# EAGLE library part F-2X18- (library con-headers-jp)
FEMALE HEADER
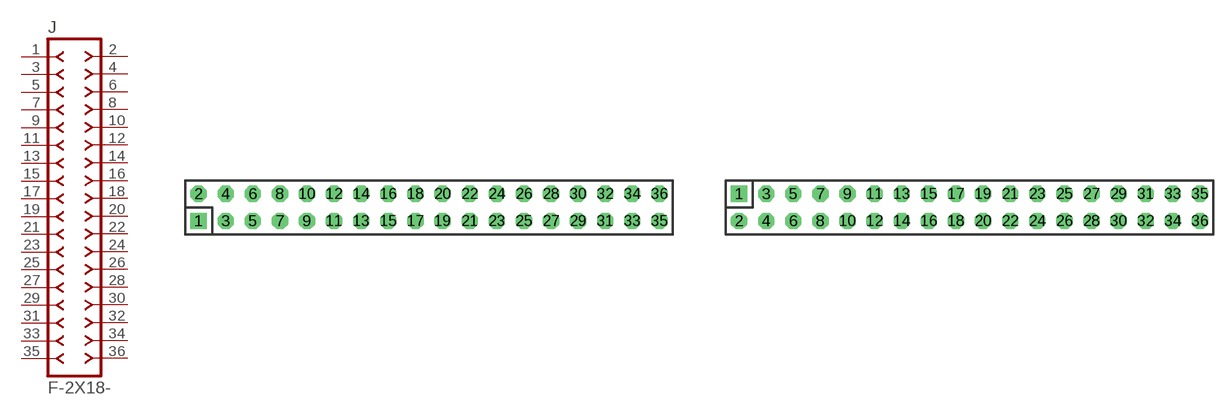
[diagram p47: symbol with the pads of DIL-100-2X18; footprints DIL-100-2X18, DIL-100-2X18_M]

Designator prefix J

## F-2X18-DIL-100  [DIL-100-2X18]
1  1  pas
2  2  pas
3  3  pas
4  4  pas
5  5  pas
6  6  pas
7  7  pas
8  8  pas
9  9  pas
10  10  pas
11  11  pas
12  12  pas
13  13  pas
14  14  pas
15  15  pas
16  16  pas
17  17  pas
18  18  pas
19  19  pas
20  20  pas
21  21  pas
22  22  pas
23  23  pas
24  24  pas
25  25  pas
26  26  pas
27  27  pas
28  28  pas
29  29  pas
30  30  pas
31  31  pas
32  32  pas
33  33  pas
34  34  pas
35  35  pas
36  36  pas

## F-2X18-DIL-100_M  [DIL-100-2X18_M]
Pads as for DIL-100-2X18

## F-2X18-DIL-2MM  [DIL-2MM-2X18]
Pads as for DIL-100-2X18

## F-2X18-DIL-2MM_M  [DIL-2MM-2X18_M]
Pads as for DIL-100-2X18

## F-2X18-71991  [71991-36]
Pads as for DIL-100-2X18

## Footprint DIL-100-2X18 (pad centres in mm)
PIN HEADER - 0.1"
drill 1.016 square: 1 -21.59,-1.27
drill 1.016 octagon: 2 -21.59,1.27; 3 -19.05,-1.27; 4 -19.05,1.27; 5 -16.51,-1.27; 6 -16.51,1.27; 7 -13.97,-1.27; 8 -13.97,1.27; 9 -11.43,-1.27; 10 -11.43,1.27; 11 -8.89,-1.27; 12 -8.89,1.27; 13 -6.35,-1.27; 14 -6.35,1.27; 15 -3.81,-1.27; 16 -3.81,1.27; 17 -1.27,-1.27; 18 -1.27,1.27; 19 1.27,-1.27; 20 1.27,1.27; 21 3.81,-1.27; 22 3.81,1.27; 23 6.35,-1.27; 24 6.35,1.27; 25 8.89,-1.27; 26 8.89,1.27; 27 11.43,-1.27; 28 11.43,1.27; 29 13.97,-1.27; 30 13.97,1.27; 31 16.51,-1.27; 32 16.51,1.27; 33 19.05,-1.27; 34 19.05,1.27; 35 21.59,-1.27; 36 21.59,1.27

## Footprint DIL-100-2X18_M (pad centres in mm)
PIN HEADER - MIRRORED 0.1"
drill 1.016 square: 1 -21.59,1.27
drill 1.016 octagon: 2 -21.59,-1.27; 3 -19.05,1.27; 4 -19.05,-1.27; 5 -16.51,1.27; 6 -16.51,-1.27; 7 -13.97,1.27; 8 -13.97,-1.27; 9 -11.43,1.27; 10 -11.43,-1.27; 11 -8.89,1.27; 12 -8.89,-1.27; 13 -6.35,1.27; 14 -6.35,-1.27; 15 -3.81,1.27; 16 -3.81,-1.27; 17 -1.27,1.27; 18 -1.27,-1.27; 19 1.27,1.27; 20 1.27,-1.27; 21 3.81,1.27; 22 3.81,-1.27; 23 6.35,1.27; 24 6.35,-1.27; 25 8.89,1.27; 26 8.89,-1.27; 27 11.43,1.27; 28 11.43,-1.27; 29 13.97,1.27; 30 13.97,-1.27; 31 16.51,1.27; 32 16.51,-1.27; 33 19.05,1.27; 34 19.05,-1.27; 35 21.59,1.27; 36 21.59,-1.27

## Footprint DIL-2MM-2X18 (pad centres in mm)
PIN HEADER - 2MM
drill 0.711 square: 1 -17,-1
drill 0.711: 2 -17,1; 3 -15,-1; 4 -15,1; 5 -13,-1; 6 -13,1; 7 -11,-1; 8 -11,1; 9 -9,-1; 10 -9,1; 11 -7,-1; 12 -7,1; 13 -5,-1; 14 -5,1; 15 -3,-1; 16 -3,1; 17 -1,-1; 18 -1,1; 19 1,-1; 20 1,1; 21 3,-1; 22 3,1; 23 5,-1; 24 5,1; 25 7,-1; 26 7,1; 27 9,-1; 28 9,1; 29 11,-1; 30 11,1; 31 13,-1; 32 13,1; 33 15,1; 34 15,-1; 35 17,1; 36 17,-1

## Footprint DIL-2MM-2X18_M (pad centres in mm)
PIN HEADER - MIRRORED 2MM
drill 0.711 square: 1 -17,1
drill 0.711: 2 -17,-1; 3 -15,1; 4 -15,-1; 5 -13,1; 6 -13,-1; 7 -11,1; 8 -11,-1; 9 -9,1; 10 -9,-1; 11 -7,1; 12 -7,-1; 13 -5,1; 14 -5,-1; 15 -3,1; 16 -3,-1; 17 -1,1; 18 -1,-1; 19 1,1; 20 1,-1; 21 3,1; 22 3,-1; 23 5,1; 24 5,-1; 25 7,1; 26 7,-1; 27 9,1; 28 9,-1; 29 11,1; 30 11,-1; 31 13,1; 32 13,-1; 33 15,-1; 34 15,1; 35 17,-1; 36 17,1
